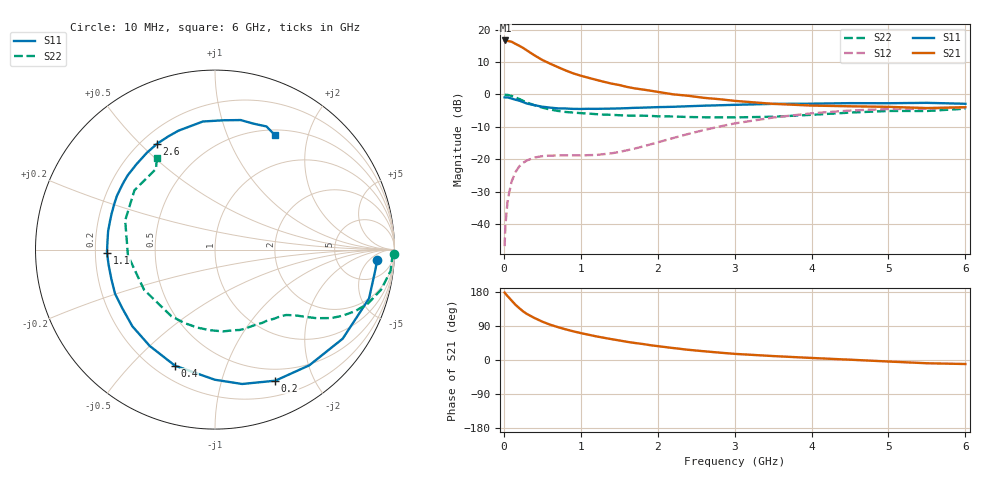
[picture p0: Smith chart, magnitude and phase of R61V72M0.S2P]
! SIEMENS Small Signal Semiconductors
! BFR193
! Si NPN RF Bipolar Junction Transistor in SOT23
! VCE = 1.75 V  IC = 2 mA
! Common Emitter S-Parameters:  May  1996
# GHz  S  MA  R  50
!  f  S11  S21  S12  S22
! GHz  MAG  ANG  MAG  ANG  MAG  ANG  MAG  ANG
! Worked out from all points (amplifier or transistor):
!   36 points, 10 MHz to 6 GHz, reference 50 ohm
!   highest |S21| = 16.7 dB at 20 MHz (marker M1)
!   |S21| within 3 dB of that: start of sweep to 295.1 MHz
!   unconditionally stable (mu >= 1): 1.147 GHz to 2.065 GHz
!   at 250 MHz: K = 0.24, MSG = 17.7 dB, |S12| = -21.1 dB
!   at 1.4 GHz: K = 1.12, MAG = 8.6 dB, |S12| = -18.1 dB
!   at 6 GHz: K = 1.00, MSG = 0.0 dB, |S12| = -3.9 dB
!   S11 on the Smith chart (normalised r, x): 10 MHz: 14, -9; 200 MHz: 0.36, -1.50; 400 MHz: 0.28, -0.68; 1.1 GHz: 0.25, -0.01; 2.6 GHz: 0.26, +0.56; 6 GHz: 0.57, +1.50
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0.01  0.9043 -3.7  6.792 178.0  0.0046 87.5  0.9967 -1.3
0.02  0.9012 -6.8  6.804 175.2  0.0095 85.7  0.9883 -2.8
0.05  0.9004 -17.6  6.682 168.3  0.0237 80.1  0.9852 -7.0
0.1  0.8675 -34.9  6.502 157.1  0.0453 71.3  0.9515 -13.6
0.15  0.8317 -50.8  6.045 146.0  0.0633 63.0  0.904 -19.4
0.2  0.804 -65.3  5.639 136.9  0.0779 56.0  0.8531 -23.7
0.25  0.7638 -78.6  5.227 128.4  0.0885 50.2  0.8002 -27.4
0.3  0.725 -90.1  4.774 121.5  0.0964 45.8  0.7537 -30.4
0.4  0.6841 -109.0  4 110.7  0.1069 39.1  0.6814 -34.1
0.5  0.6484 -124.1  3.405 101.2  0.1122 34.6  0.6285 -36.6
0.6  0.6281 -137.1  2.995 93.4  0.1143 32.5  0.587 -38.8
0.7  0.6112 -147.7  2.65 86.9  0.1152 31.6  0.559 -40.8
0.9  0.6003 -164.0  2.12 75.8  0.1158 32.0  0.5266 -44.5
1.1  0.6022 -178.2  1.809 66.7  0.1163 36.2  0.5076 -49.2
1.3  0.6042 170.3  1.57 58.7  0.1205 42.5  0.49 -54.1
1.6  0.6157 155.9  1.309 48.0  0.1381 52.2  0.4743 -63.1
2.2  0.6464 132.5  1.006 31.6  0.2131 61.3  0.458 -84.5
2.6  0.6723 118.7  0.888 23.1  0.2829 59.3  0.4457 -102.5
3.5  0.7169 95.4  0.718 10.4  0.4414 43.7  0.4543 -150.5
4.5  0.7358 78.8  0.658 0.8  0.5662 23.1  0.5261 162.0
5.5  0.7437 67.3  0.618 -8.6  0.6018 4.4  0.5569 126.2
6  0.7198 62.4  0.637 -10.6  0.6351 -0.8  0.6038 122.4
